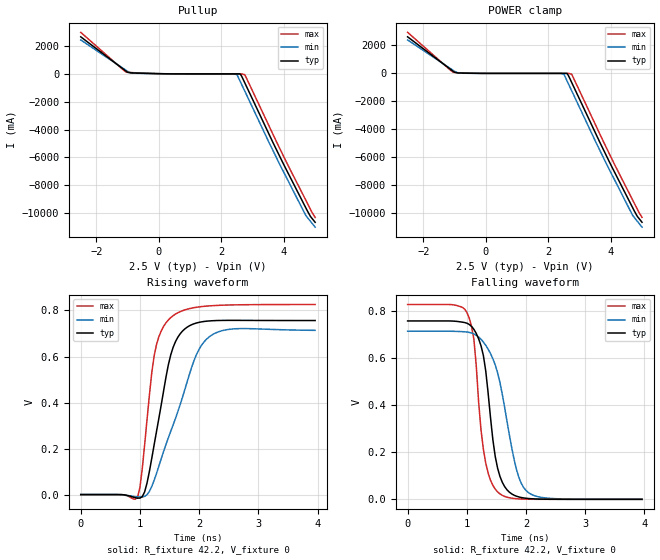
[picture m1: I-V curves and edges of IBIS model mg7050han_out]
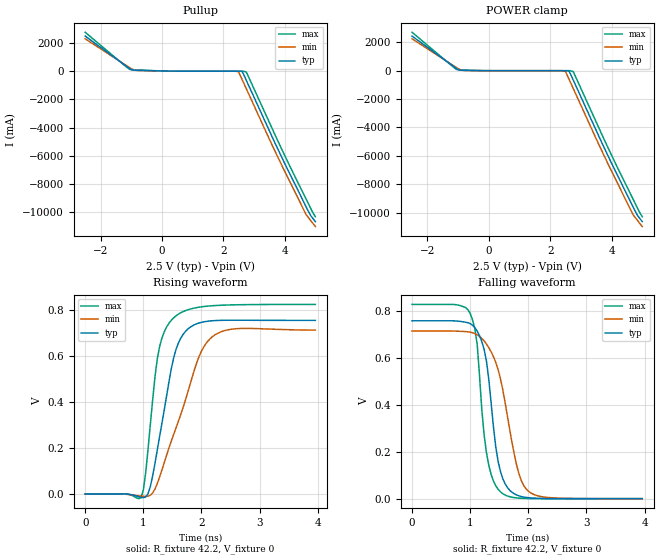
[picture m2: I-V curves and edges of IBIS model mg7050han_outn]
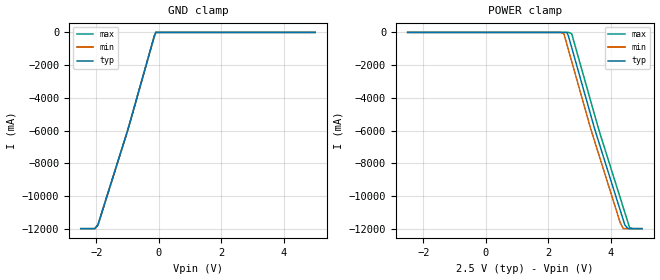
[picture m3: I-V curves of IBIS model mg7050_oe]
|   IBIS File mg7050han_4a_25v_85.ibs  ZSEL=L(ZO=85ohm)
[IBIS Ver]   3.2
[Comment Char]   |_char
[File name]   mg7050han_4a_25v_85.ibs
[File Rev]   1.0
[Date]   Jan 23, 2014
[Source]
|   Component MG7050HAN HCSL 4-OUTPUT 2.5V
[Component]   mg7050han-hcsl-4out-85ohm
[Manufacturer]   Seiko Epson Corporation
[Package]
| variable   typ   min   max
R_pkg   0.27   NA   NA
L_pkg   1.66n   NA   NA
C_pkg   0.53p   NA   NA
[Pin]   signal_name   model_name   R_pin   L_pin   C_pin
1   vcc1   POWER   NA   NA   NA
2   out1p   mg7050han_out   0.34   2.1nH   0.58pF
3   out1n   mg7050han_outn  0.25   1.5nH   0.50pF
4   out2p   mg7050han_out   0.22   1.3nH   0.44pF
5   out2n   mg7050han_outn  0.25   1.7nH   0.59pF
6   zsel   mg7050_zsel   NA   NA   NA
7   oe   mg7050_oe   NA   NA   NA
8   out3n   mg7050han_outn  0.25   1.7nH   0.62pF
9   out3p   mg7050han_out   0.22   1.3nH   0.49pF
10   out4n   mg7050han_outn  0.25   1.5nH   0.46pF
11   out4p   mg7050han_out   0.34   2.1nH   0.57pF
12   vcc2   POWER   NA   NA   NA
13   vcc   POWER   NA   NA   NA
14   gnd   GND   NA   NA   NA
[Diff Pin] inv_pin vdiff   tdelay_typ
2   3   0   0
4   5   0   0
9   8   0   0
11   10   0   0
| Models and submodels in the file (4): mg7050han_out (Open_source), mg7050han_outn (Open_source), mg7050_oe (Input), mg7050_zsel (Input)
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[Model]   mg7050han_out
Model_type Open_source
Enable Active-High
Polarity Non-Inverting
Vref=0
Vmeas=0.375
Rref=42.2
Cref=0
C_comp   4.96p   7.43p   5.19p
[Temperature Range] 25   85   -40
[Voltage Range]   2.5   2.375   2.625
[POWER Clamp Reference]2.5   2.375   2.625
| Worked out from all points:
|   slope of the pullup table from 0 to 0.375 V, typ, clamps not added: 29.5 ohm
|   POWER clamp passes 1 mA (typ) near -0.15 V on its own axis
|   falling waveform, R_fixture 42.2, V_fixture 0: 20-80 % time 222ps typ, 345ps min, 186ps max; typ from 0.756 V to 0 V
|   rising waveform, R_fixture 42.2, V_fixture 0: 20-80 % time 323ps typ, 555ps min, 231ps max; typ from 0 V to 0.756 V
[Pullup]
-2.5V     2.639A     2.416A     2.962A
-1.05V    176.3mA    242.4mA    117.6mA
-900mV    58.16mA    58.89mA    78.4mA
-750mV    44.92mA    31.73mA    64.06mA
2.4V      -17.99mA   -17.16mA   -19.68mA
2.5V      -17.99mA   -72.75mA   -19.69mA
2.6V      -17.99mA   -545mA     -19.69mA
2.75V     -664.2mA   -1.257A    -74.54mA
3.8V      -5.622A    -6.194A    -5.051A
4.7V      -9.608A    -10.15A    -9.061A
4.85V     -10.23A    -10.58A    -9.719A
5V        -10.65A    -11A       -10.3A
[POWER Clamp]
-2.5V     2.61A      2.389A     2.933A
-1.05V    157.6mA    226.1mA    90.16mA
-900mV    32.6mA     39.46mA    48.3mA
-750mV    21.93mA    12.82mA    37.42mA
2.4V      -194.4pA   -217pA     -182.9pA
2.5V      -205.6pA   -60.77mA   -194.1pA
2.6V      -216.8pA   -533.9mA   -205.3pA
2.75V     -652.5mA   -1.246A    -60.77mA
3.8V      -5.61A     -6.183A    -5.038A
4.7V      -9.596A    -10.14A    -9.048A
4.85V     -10.22A    -10.57A    -9.706A
5V        -10.64A    -10.98A    -10.29A
[Falling Waveform]
R_fixture=42.2
V_fixture=0
V_fixture_min=0
V_fixture_max=0
0s        756.4mV    713mV      826.1mV
1ns       747mV      709.6mV    793.3mV
1.12ns    720.6mV    700.9mV    678mV
1.24ns    651mV      678.7mV    293.6mV
1.32ns    543.8mV    653.1mV    153.6mV
1.44ns    252.9mV    596.2mV    59.31mV
1.56ns    97.13mV    494.9mV    23.06mV
1.84ns    13.14mV    125.8mV    2.564mV
2.04ns    3.494mV    28.87mV    551.3uV
3.96ns    0V         8.06uV     0V
[Rising Waveform]
R_fixture=42.2
V_fixture=0
V_fixture_min=0
V_fixture_max=0
0s        0V         850.3nV    0V
960ps     -15.6mV    -10.12mV   -12.11mV
1ns       -15.34mV   -10.63mV   31.92mV
1.08ns    12.34mV    -7.733mV   217.9mV
1.24ns    216.5mV    62.14mV    603.1mV
1.36ns    390.5mV    156.1mV    711.5mV
1.56ns    639.4mV    302.6mV    777.4mV
1.96ns    746mV      611.5mV    814.1mV
2.2ns     755.1mV    690.9mV    820.5mV
3.96ns    756.3mV    713.7mV    826mV
[Ramp]
R_load=42.2
dV/dt_r   4.538E-1/3.227E-10   4.278E-1/5.534E-10   4.957E-1/2.289E-10
dV/dt_f   4.538E-1/2.193E-10   4.278E-1/3.441E-10   4.957E-1/1.825E-10
|[End   mg7050han_out
[Model]   mg7050han_outn
Model_type Open_source
Enable Active-High
Polarity Inverting
Vref=0
Vmeas=0.375
Rref=42.2
Cref=0
C_comp   4.96p   7.43p   5.19p
[Temperature Range] 25   85   -40
[Voltage Range]   2.5   2.375   2.625
[POWER Clamp Reference]2.5   2.375   2.625
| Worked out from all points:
|   slope of the pullup table from 0 to 0.375 V, typ, clamps not added: 29.5 ohm
|   POWER clamp passes 1 mA (typ) near -0.15 V on its own axis
|   falling waveform, R_fixture 42.2, V_fixture 0: 20-80 % time 223ps typ, 347ps min, 185ps max; typ from 0.756 V to 0 V
|   rising waveform, R_fixture 42.2, V_fixture 0: 20-80 % time 322ps typ, 550ps min, 231ps max; typ from 0 V to 0.756 V
[Pullup]
-2.5V     2.461A     2.271A     2.731A
-1.05V    164.5mA    228mA      113.7mA
-900mV    57.87mA    57.73mA    78.22mA
-750mV    44.85mA    31.68mA    63.93mA
2.4V      -17.99mA   -17.16mA   -19.68mA
2.5V      -17.99mA   -72.75mA   -19.69mA
2.6V      -17.99mA   -545mA     -19.69mA
2.75V     -664.2mA   -1.257A    -74.54mA
3.8V      -5.622A    -6.194A    -5.051A
4.7V      -9.608A    -10.15A    -9.061A
4.85V     -10.23A    -10.58A    -9.719A
5V        -10.65A    -11A       -10.3A
[POWER Clamp]
-2.5V     2.435A     2.246A     2.705A
-1.05V    147mA      212.6mA    86.61mA
-900mV    32.41mA    38.61mA    48.16mA
-750mV    21.89mA    12.8mA     37.31mA
2.4V      -194.4pA   -217pA     -182.9pA
2.5V      -205.6pA   -60.77mA   -194.1pA
2.6V      -216.8pA   -533.9mA   -205.3pA
2.75V     -652.5mA   -1.246A    -60.77mA
3.8V      -5.61A     -6.183A    -5.038A
4.7V      -9.596A    -10.14A    -9.048A
4.85V     -10.22A    -10.57A    -9.706A
5V        -10.64A    -10.98A    -10.29A
[Falling Waveform]
R_fixture=42.2
V_fixture=0
V_fixture_min=0
V_fixture_max=0
0s        756.3mV    713mV      826.1mV
1ns       744.3mV    708.2mV    787.4mV
1.12ns    712.8mV    696.9mV    656.7mV
1.2ns     668.1mV    681.5mV    376.8mV
1.28ns    584.8mV    657.5mV    195.4mV
1.44ns    219.9mV    579.3mV    54.92mV
1.52ns    116.1mV    510.9mV    29.27mV
1.8ns     15.46mV    141.4mV    3.252mV
2ns       4.092mV    32.09mV    694.2uV
3.96ns    0V         7.362uV    0V
[Rising Waveform]
R_fixture=42.2
V_fixture=0
V_fixture_min=0
V_fixture_max=0
0s        1.266uV    2.559uV    0V
960ps     -14.84mV   -9.481mV   -16.74mV
1.04ns    -13.2mV    -10.6mV    91.35mV
1.12ns    31.98mV    -5.641mV   301.2mV
1.2ns     132.9mV    21.74mV    508.8mV
1.28ns    250.3mV    73.54mV    642.3mV
1.56ns    627.9mV    286.3mV    775.8mV
1.96ns    745.1mV    599.5mV    813.9mV
2.2ns     754.9mV    687.4mV    820.4mV
3.96ns    756.3mV    713.8mV    826mV
[Ramp]
R_load=42.2
dV/dt_r   4.538E-1/3.210E-10   4.278E-1/5.496E-10   4.957E-1/2.285E-10
dV/dt_f   4.538E-1/2.199E-10   4.278E-1/3.461E-10   4.957E-1/1.827E-10
|[End   mg7050han_outn
[Model]   mg7050_oe
Model_type Input
Vinh=1.75
Vinl=0.75
C_comp   3p   3p   3p
[Temperature Range] 25   85   -40
[Voltage Range]   2.5   2.375   2.625
[POWER Clamp Reference]2.5   2.375   2.625
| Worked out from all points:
|   GND clamp passes 1 mA (typ) near -0.10 V on its own axis
[GND Clamp]
-2.5V     -12A       -12A       -12A
-2.05V    -12A       -12A       -12A
-1.95V    -11.77A    -11.77A    -11.77A
-1V       -6A        -6A        -6A
-150mV    -254mA     -254mA     -254mA
-100mV    -25.23uA   -23.33uA   -29.37uA
5V        24.28uA    24.81uA    25.61uA
[POWER Clamp]
-2.5V     24.28uA    23.63uA    26.96uA
2.4V      -23.29uA   -22.62uA   -25.87uA
2.5V      -24.26uA   -84.67mA   -26.95uA
2.6V      -25.23uA   -761.8mA   -28.02uA
2.75V     -931.1mA   -1.778A    -84.67mA
3.35V     -4.994A    -5.84A     -4.148A
3.5V      -6A        -6.759A    -5.163A
4.3V      -10.86A    -11.62A    -10.1A
4.4V      -11.47A    -12A       -10.71A
4.45V     -11.77A    -12A       -11.01A
4.6V      -12A       -12A       -11.92A
5V        -12A       -12A       -12A
